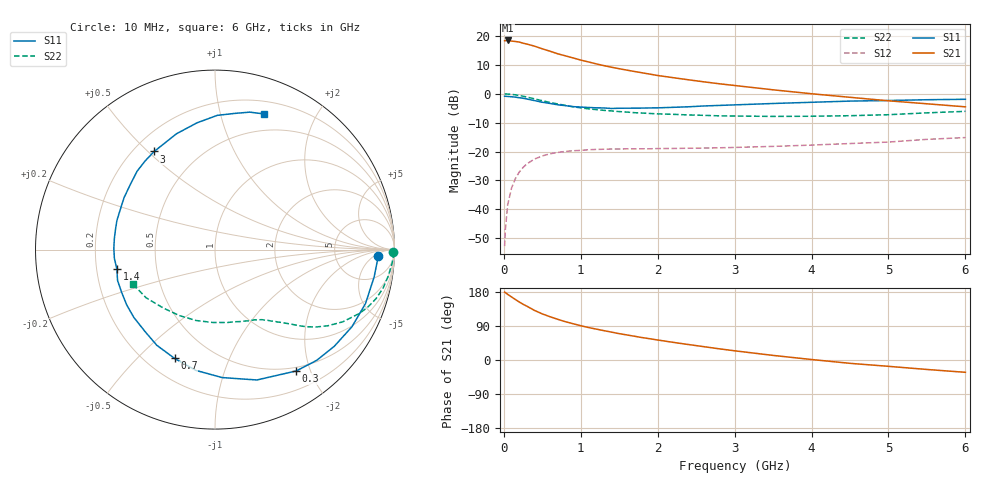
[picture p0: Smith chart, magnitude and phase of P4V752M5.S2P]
! SIEMENS Small Signal Semiconductors
! BFP182
! Si NPN RF Bipolar Junction Transistor in SOT143
! VCE = 0.75 V  IC = 2.5 mA
! Common Emitter S-Parameters:  March  1996
# GHz  S  MA  R  50
!  f  S11  S21  S12  S22
! GHz  MAG  ANG  MAG  ANG  MAG  ANG  MAG  ANG
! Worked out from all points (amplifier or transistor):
!   36 points, 10 MHz to 6 GHz, reference 50 ohm
!   highest |S21| = 18.5 dB at 50 MHz (marker M1)
!   |S21| within 3 dB of that: start of sweep to 512.7 MHz
!   unconditionally stable (mu >= 1): 1.902 GHz to end of sweep
!   at 250 MHz: K = 0.15, MSG = 21.5 dB, |S12| = -25.5 dB
!   at 1.4 GHz: K = 0.77, MSG = 14.2 dB, |S12| = -19.1 dB
!   at 6 GHz: K = 1.14, MAG = 3.0 dB, |S12| = -15.2 dB
!   S11 on the Smith chart (normalised r, x): 10 MHz: 18, -7; 300 MHz: 0.45, -1.79; 700 MHz: 0.31, -0.65; 1.4 GHz: 0.29, -0.09; 3 GHz: 0.28, +0.52; 6 GHz: 0.32, +1.38
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0.01  0.9076 -2.1  8.299 179.0  0.0023 86.7  0.9933 -0.9
0.02  0.9069 -3.9  8.325 177.9  0.0045 85.3  0.9951 -1.8
0.05  0.8997 -9.8  8.395 173.2  0.012 85.2  0.9893 -4.4
0.1  0.8907 -19.8  8.193 166.4  0.0233 78.3  0.9762 -8.8
0.15  0.8757 -29.4  8.055 159.6  0.0341 73.4  0.9604 -13.0
0.2  0.8556 -39.0  7.883 153.1  0.0441 68.3  0.9375 -17.0
0.3  0.8136 -56.2  7.268 141.9  0.0613 58.9  0.8801 -23.8
0.4  0.7629 -72.2  6.676 130.7  0.0744 51.0  0.8175 -29.5
0.5  0.7141 -86.8  6.016 121.7  0.084 44.0  0.7587 -34.0
0.6  0.6813 -99.0  5.468 114.2  0.0916 38.8  0.7099 -37.4
0.7  0.6466 -110.4  4.933 107.4  0.0965 34.6  0.667 -40.1
0.8  0.6239 -121.3  4.545 101.1  0.1007 31.0  0.63 -42.3
0.9  0.6001 -130.6  4.182 95.7  0.1033 28.0  0.5965 -44.2
1.1  0.5805 -147.9  3.566 85.7  0.1075 23.2  0.5494 -47.6
1.4  0.5573 -168.9  2.885 73.6  0.1106 18.1  0.5058 -51.9
1.8  0.5661 167.9  2.307 59.1  0.1118 15.2  0.4642 -57.3
2.2  0.5835 150.3  1.904 46.6  0.1131 13.1  0.4414 -63.8
3  0.6433 121.8  1.394 24.3  0.1179 11.8  0.4124 -79.9
3.5  0.68 108.4  1.173 12.1  0.1229 11.8  0.4063 -91.6
4.5  0.7481 89.0  0.87 -8.8  0.1377 11.1  0.4179 -118.5
5.5  0.79 75.8  0.672 -25.0  0.1627 9.6  0.4684 -145.0
6  0.8041 70.0  0.595 -32.5  0.1747 6.4  0.4969 -157.4
